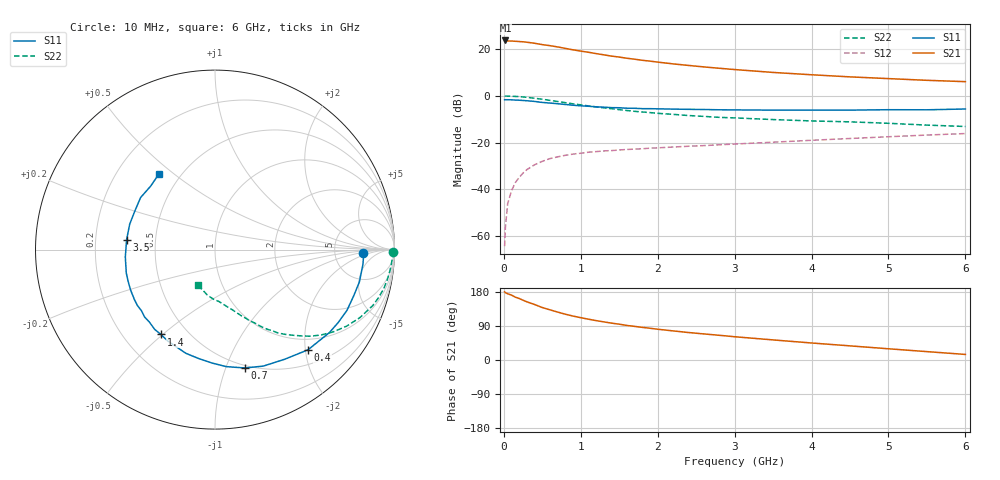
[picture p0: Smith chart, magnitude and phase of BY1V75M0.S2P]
! SIEMENS Small Signal Semiconductors
! BFY420
! Si NPN RF SIEGET Grounded Emitter Transistor in MICRO-X
! VCE = 1.75 V  IC = 5 mA
! Common Emitter S-Parameters:  October  1996
# GHz  S  MA  R  50
!  f  S11  S21  S12  S22
! GHz  MAG  ANG  MAG  ANG  MAG  ANG  MAG  ANG
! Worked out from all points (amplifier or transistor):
!   36 points, 10 MHz to 6 GHz, reference 50 ohm
!   highest |S21| = 23.8 dB at 20 MHz (marker M1)
!   |S21| within 3 dB of that: start of sweep to 735.4 MHz
!   unconditionally stable (mu >= 1): 3.131 GHz to end of sweep
!   at 250 MHz: K = 0.10, MSG = 28.1 dB, |S12| = -33.1 dB
!   at 1.4 GHz: K = 0.54, MSG = 20.3 dB, |S12| = -23.5 dB
!   at 6 GHz: K = 1.15, MAG = 8.8 dB, |S12| = -16.1 dB
!   S11 on the Smith chart (normalised r, x): 10 MHz: 10, -1; 400 MHz: 0.77, -2.05; 700 MHz: 0.48, -1.17; 1.4 GHz: 0.36, -0.49; 3.5 GHz: 0.34, +0.05; 6 GHz: 0.38, +0.44
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0.01  0.8273 -1.5  15.39 179.8  0.0006 92.5  0.9901 -0.7
0.02  0.8283 -2.8  15.46 177.7  0.0015 80.4  0.9932 -1.3
0.05  0.8283 -5.8  15.07 174.8  0.0049 88.7  0.9887 -3.3
0.1  0.8244 -12.6  15.01 171.2  0.0093 83.3  0.9823 -6.7
0.15  0.8148 -18.3  14.84 165.8  0.0139 78.5  0.9743 -10.1
0.25  0.7977 -30.6  14.45 157.7  0.0222 74.4  0.9495 -16.4
0.3  0.7876 -35.9  14.16 153.5  0.0263 71.7  0.933 -19.5
0.4  0.7618 -47.1  13.45 146.4  0.0334 65.9  0.8915 -25.2
0.5  0.7241 -57.5  12.59 138.4  0.0396 61.3  0.8482 -30.2
0.6  0.7026 -67.5  11.95 132.4  0.0453 57.3  0.803 -34.8
0.7  0.68 -75.9  11.22 126.4  0.0494 53.5  0.7591 -38.8
0.9  0.6317 -91.7  9.727 115.9  0.0566 47.6  0.6771 -45.2
1.1  0.6001 -105.7  8.624 107.7  0.0621 43.6  0.6105 -50.6
1.4  0.5606 -122.5  7.133 97.3  0.0672 39.7  0.5322 -56.6
1.6  0.5445 -132.3  6.418 91.2  0.0711 38.0  0.4865 -60.0
1.8  0.5329 -140.3  5.81 86.1  0.0736 36.7  0.453 -62.7
2.2  0.5214 -154.4  4.863 76.8  0.0801 35.0  0.4022 -67.8
2.8  0.5041 -170.4  3.916 65.2  0.0895 33.5  0.347 -74.2
3.5  0.4956 173.6  3.187 53.0  0.1018 31.7  0.311 -80.7
4.5  0.4956 154.3  2.56 37.3  0.1222 27.8  0.2779 -91.1
5.5  0.5037 135.2  2.16 22.1  0.1448 22.1  0.2366 -106.4
6  0.5243 126.7  2.021 14.7  0.1559 18.8  0.2209 -116.1
